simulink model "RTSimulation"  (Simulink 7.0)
settings: Solver=FixedStepDiscrete  StartTime=0.0  StopTime=inf  RelTol=1e-3
PreLoadFcn:
  | initialize;
  | scramInitialize;
InitFcn:
  | dirName = [bdroot '_xpc_rtw'];
  | if ~isdir(dirName)
  | 	mkdir(dirName);
  | end
  | copyfile('Actuator.obj', dirName);
  | copyfile('Act2Tbl.obj', dirName);
  | copyfile('Tbl2Act.obj', dirName);
  | copyfile('xfmlib.obj', dirName);
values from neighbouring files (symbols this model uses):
  acal = acal(:)    [initialize.m]
  actParams = [	bulkModulus   * pressCanon    [initialize.m]
  atype = ones(nact, 1)    [dampmatrix.m]    (also in displA2T.m = []; displEnvelope.m = varargin{1}{6}; displJacobian.m; displT2A.m = [])
  controlPeriod = 1/2048    (= 0.00048828125)    [initialize.m]
  dcal = dcal(:)    [initialize.m]
  fcal = fcal(:)    [initialize.m]
  forceCanon = 0.00444822    [initialize.m]
  inertia = inertia + inertiaP2Q([0 0 0], massA(i), cgA(:,i)-cg,  									inertiaCanon, massCanon)    [initialize.m]
  inertiaMask = zeros(3, 1)    [initialize.m]
  lengthCanon = 25.4    [initialize.m]
  mass = ones(3, 1) * (sum(massA) + massT + massS)    [initialize.m]
  massMask = zeros(3, 1)    [initialize.m]
  nAdcU = 6    [initialize.m]
  node = scgtnodestruct(node)    [scramInitialize.m]
  nTbl = length(dof)    [initialize.m]
  returnPress = 50    [initialize.m]
  rtg = cg    [initialize.m]
  samplePeriod = controlPeriod/upsampleFactor    (= 0.00048828125)    [initialize.m]    (also in viewer.m = eval(getHeaderValue(header, 'DELTA_T')))
  staticForce = forceT2A(ftbl, dtbl0, dof, rh, rb, rl, canon, atype)    [initialize.m]
  x = []    [loadbin.m]    (also in quake.m = 365; viewer.m = 40; player.m = xPanel + panelWide + margin; resondemo.m = xOrigin + marginWide + panelWide + plotMarginWide)
undefined symbols (not defined in the file or in its folder): animation, DiscIntNeverNeededParam, friction, yieldDispl
libraries: LibDynamics x12, LibTransforms x12, cwcec_scgtLib x3, xpclib x3

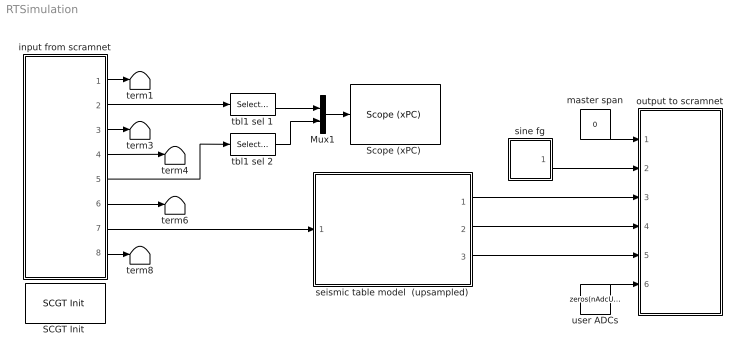
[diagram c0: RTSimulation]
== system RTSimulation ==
  Mux1 : Mux  Inputs=2
  "SCGT Init " : cwcec_scgtLib/SCGT Init   node=node  pci=-1
  "Scope (xPC) " : xpclib/Misc./Scope (xPC)   SystemSampleTime=-1  scopeno=1  scopetype=Target  autostart=on  viewmode=Graphical redraw  formatstr='%15.6f'  grid=on  ylimits=[0,0]  nosamples=1024  noprepostsamples=0  interleave=1  triggermode=FreeRun  triggersignal=1  triggerlevel=0.0  triggerslope=Either  triggerscope=1  triggersample=0  filename=data.dat  mode=Lazy  writesize=512  autorestart=off
  input from scramnet : Subsystem
  master span : Constant  Value=0  OutDataType=sfix(16)  OutScaling=2^0
  output to scramnet : Subsystem
  seismic table model  (upsampled) : Subsystem  TreatAsAtomicUnit=on
  sine fg : Subsystem  mask(Sine Function Generator){id=x, ampl=0.3, freq=4, phase=0, spanInterval=1, samplePeriod=controlPeriod}
      mask prompts: id "DOF"; ampl "Amplitude"; freq "Frequency (Hz)"; phase "Phase (deg)"; spanInterval "Span interval (sec)"; samplePeriod "Sample period (sec)"
  tbl1 sel 1 : Selector  IndexOptions=Index vector (dialog)  Indices=1  OutputSizes=1
  tbl1 sel 2 : Selector  IndexOptions=Index vector (dialog)  Indices=1  OutputSizes=1
  term{1,3..4,6,8} (5 alike) : Terminator
  user ADCs : Constant  Value=zeros(nAdcU, 1)  OutDataType=sfix(16)  OutScaling=2^0
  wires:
  input from scramnet/1(master span) -> term1/1
  input from scramnet/3(displ fbk) -> term3/1
  input from scramnet/4(veloc fbk) -> term4/1
  input from scramnet/6(force fbk) -> term6/1
  input from scramnet/8(user adcs) -> term8/1
  Mux1/1 -> "Scope (xPC) "/1
  input from scramnet/2(ref) -> tbl1 sel 1/1
  input from scramnet/5(accel fbk) -> tbl1 sel 2/1
  tbl1 sel 1/1 -> Mux1/1
  tbl1 sel 2/1 -> Mux1/2
  user ADCs/1 -> output to scramnet/6(user adcs)
  master span/1 -> output to scramnet/1(master span)
  input from scramnet/7(valve cmd) -> seismic table model  (upsampled)/1(valve cmd)
  sine fg/1(out) -> output to scramnet/2(ref)
  seismic table model  (upsampled)/1(displ) -> output to scramnet/3(displ fbk)
  seismic table model  (upsampled)/2(accel) -> output to scramnet/4(accel fbks)
  seismic table model  (upsampled)/3(force) -> output to scramnet/5(force fbk)

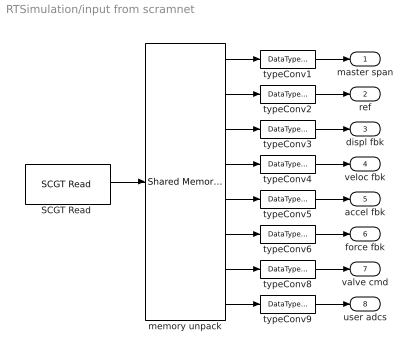
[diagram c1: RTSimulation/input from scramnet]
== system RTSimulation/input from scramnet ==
  "SCGT Read " : cwcec_scgtLib/SCGT Read   partition=node.Partitions(7:14)  ts=controlPeriod  pci=-1
  memory unpack : xpclib/Shared Memory/Shared Memory Unpack   partition=node.Partitions(7:14)
  typeConv{1..6,8..9} (8 alike) : DataTypeConversion  OutDataTypeMode=double  OutDataType=sfix(16)  OutScaling=2^0
  master span : Outport  OutDataType=sfix(16)  OutScaling=2^0
  ref : Outport  Port=2  OutDataType=sfix(16)  OutScaling=2^0
  displ fbk : Outport  Port=3  OutDataType=sfix(16)  OutScaling=2^0
  veloc fbk : Outport  Port=4  OutDataType=sfix(16)  OutScaling=2^0
  accel fbk : Outport  Port=5  OutDataType=sfix(16)  OutScaling=2^0
  force fbk : Outport  Port=6  OutDataType=sfix(16)  OutScaling=2^0
  valve cmd : Outport  Port=7  OutDataType=sfix(16)  OutScaling=2^0
  user adcs : Outport  Port=8  OutDataType=sfix(16)  OutScaling=2^0
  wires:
  "SCGT Read "/1 -> memory unpack/1
  typeConv1/1 -> master span/1
  typeConv2/1 -> ref/1
  typeConv3/1 -> displ fbk/1
  typeConv4/1 -> veloc fbk/1
  typeConv5/1 -> accel fbk/1
  typeConv6/1 -> force fbk/1
  typeConv8/1 -> valve cmd/1
  typeConv9/1 -> user adcs/1
  memory unpack/1 -> typeConv1/1
  memory unpack/8 -> typeConv9/1
  memory unpack/2 -> typeConv2/1
  memory unpack/7 -> typeConv8/1
  memory unpack/3 -> typeConv3/1
  memory unpack/4 -> typeConv4/1
  memory unpack/5 -> typeConv5/1
  memory unpack/6 -> typeConv6/1

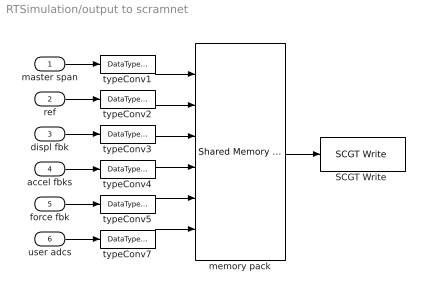
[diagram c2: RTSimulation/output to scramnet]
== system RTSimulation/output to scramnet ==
  master span : Inport  OutDataType=sfix(16)  OutScaling=2^0
  ref : Inport  Port=2  OutDataType=sfix(16)  OutScaling=2^0
  displ fbk : Inport  Port=3  OutDataType=sfix(16)  OutScaling=2^0
  accel fbks : Inport  Port=4  OutDataType=sfix(16)  OutScaling=2^0
  force fbk : Inport  Port=5  OutDataType=sfix(16)  OutScaling=2^0
  user adcs : Inport  Port=6  OutDataType=sfix(16)  OutScaling=2^0
  "SCGT Write " : cwcec_scgtLib/SCGT Write   partition=node.Partitions(1:6)  ts=controlPeriod  pci=-1
  memory pack : xpclib/Shared Memory/Shared Memory Pack   partition=node.Partitions(1:6)
  typeConv{1..5,7} (6 alike) : DataTypeConversion  OutDataTypeMode=single  OutDataType=sfix(16)  OutScaling=2^0
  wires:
  master span/1 -> typeConv1/1
  ref/1 -> typeConv2/1
  displ fbk/1 -> typeConv3/1
  accel fbks/1 -> typeConv4/1
  memory pack/1 -> "SCGT Write "/1
  typeConv1/1 -> memory pack/1
  typeConv2/1 -> memory pack/2
  typeConv3/1 -> memory pack/3
  typeConv4/1 -> memory pack/4
  force fbk/1 -> typeConv5/1
  user adcs/1 -> typeConv7/1
  typeConv5/1 -> memory pack/5
  typeConv7/1 -> memory pack/6

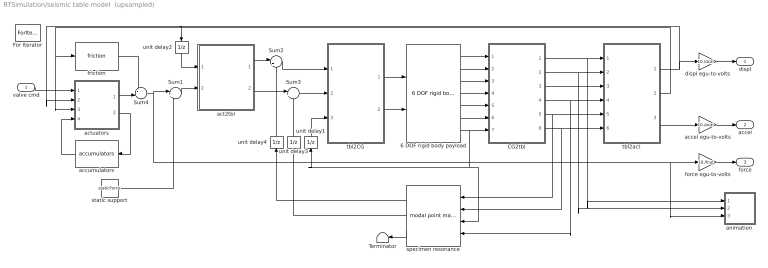
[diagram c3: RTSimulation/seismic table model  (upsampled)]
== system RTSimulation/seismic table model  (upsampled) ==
  valve cmd : Inport  OutDataType=sfix(16)  OutScaling=2^0
  6 DOF rigid body payload : LibDynamics/6 DOF rigid body payload  SystemSampleTime=-1  mass=mass.*massMask  inertia=diag(inertia.*inertiaMask)  gee=gee  massCanon=massCanon  inertiaCanon=inertiaCanon  linVelocCanon=linVelocCanon  linAccelCanon=linAccelCanon  rotDisplCanon=rotDisplCanon  rotVelocCanon=rotVelocCanon  rotAccelCanon=rotAccelCanon  rotForceCanon=rotForceCanon  initialPosition=zeros(6,1)  samplePeriod=samplePeriod
  CG2tbl : Subsystem  mask{ofst=-rtg}
      mask prompts: ofst "Origin offset"
  For Iterator : ForIterator  IterationLimit=upsampleFactor  ShowIterationPort=off
  Sum1 : Sum  Inputs=|++  OutDataType=sfix(16)  OutScaling=2^0
  Sum2 : Sum  Inputs=|+-  OutDataType=sfix(16)  OutScaling=2^0
  Sum3 : Sum  Inputs=|+-  OutDataType=sfix(16)  OutScaling=2^0
  Sum4 : Sum  Inputs=-+|  OutDataType=sfix(16)  OutScaling=2^0
  Terminator : Terminator
  accel egu-to-volts : Gain  Gain=10./acal  ParameterDataType=sfix(16)  ParameterScaling=2^0  OutDataType=sfix(16)  OutScaling=2^0
  accumulators : LibDynamics/accumulators  Orientation=left  SystemSampleTime=-1  pumpFlow=pumpFlow  supplyPressure=supplyPress  precharge=precharge  bottleVolume=volume  gasConstant=gasConstant  flowCanon=flowCanon  volumeCanon=volumeCanon  samplePeriod=samplePeriod
  act2tbl : Subsystem
  actuators : Subsystem
  animation : Subsystem  mask{azim=-37.5, elev=35, params=animation, decim=ceil((1/samplePeriod)/32), samplePeriod=-1}
      mask prompts: azim "View azimuth (degrees)"; elev "View elevation (degrees)"; params "Parameters"; decim "Decimation factor"; samplePeriod "Sample period (sec)"
  displ egu-to-volts : Gain  Gain=10./dcal  ParameterDataType=sfix(16)  ParameterScaling=2^0  OutDataType=sfix(16)  OutScaling=2^0
  force egu-to-volts : Gain  Gain=10./fcal  ParameterDataType=sfix(16)  ParameterScaling=2^0  OutDataType=sfix(16)  OutScaling=2^0
  friction : LibDynamics/friction  SystemSampleTime=-1  friction=friction * forceCanon  yieldDispl=yieldDispl * lengthCanon  hysteresis=0  velocCanon=linVelocCanon  samplePeriod=samplePeriod
  specimen resonance : LibDynamics/modal point mass  Orientation=left  SystemSampleTime=-1  mass=modalMass  freq=modalFreq  damp=modalDamp  ofst=modalCG  gee=gee  massCanon=massCanon  linAccelCanon=linAccelCanon  rotDisplCanon=rotDisplCanon  rotVelocCanon=rotVelocCanon  rotForceCanon=rotForceCanon  samplePeriod=samplePeriod
  static support : Constant  Value=staticForce  OutDataType=sfix(16)  OutScaling=2^0
  tbl2CG : Subsystem  mask{ofst=rtg}
      mask prompts: ofst "Origin offset"
  tbl2act : Subsystem
  unit delay1 : UnitDelay  Orientation=up  X0=eye(3)  SampleTime=-1
  unit delay2 : UnitDelay  Orientation=down  SampleTime=-1
  unit delay3 : UnitDelay  Orientation=up  SampleTime=-1
  unit delay4 : UnitDelay  Orientation=up  SampleTime=-1
  displ : Outport  OutDataType=sfix(16)  OutScaling=2^0
  accel : Outport  Port=2  OutDataType=sfix(16)  OutScaling=2^0
  force : Outport  Port=3  OutDataType=sfix(16)  OutScaling=2^0
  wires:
  specimen resonance/3 -> Terminator/1
  static support/1 -> Sum1/2
  Sum1/1 -> act2tbl/2(force act)
  accel egu-to-volts/1 -> accel/1
  displ egu-to-volts/1 -> displ/1
  force egu-to-volts/1 -> force/1
  accumulators/1 -> actuators/4(press)
  actuators/2(flow) -> accumulators/1
  tbl2CG/2(force rpw) -> 6 DOF rigid body payload/2
  tbl2act/1(displ act) -> displ egu-to-volts/1, actuators/2(displ), unit delay2/1
  valve cmd/1 -> actuators/1(cmds)
  tbl2CG/1(force xyz) -> 6 DOF rigid body payload/1
  6 DOF rigid body payload/1 -> CG2tbl/1(displ xyz)
  6 DOF rigid body payload/2 -> CG2tbl/2(displ rpw)
  6 DOF rigid body payload/3 -> CG2tbl/3(veloc xyz)
  6 DOF rigid body payload/4 -> CG2tbl/4(veloc rpw)
  6 DOF rigid body payload/5 -> CG2tbl/5(accel xyz)
  6 DOF rigid body payload/6 -> CG2tbl/6(accel rpw)
  6 DOF rigid body payload/7 -> specimen resonance/3, unit delay1/1, CG2tbl/7(DCM)
  tbl2act/3(accel act) -> accel egu-to-volts/1
  unit delay1/1 -> tbl2CG/3(DCM)
  unit delay2/1 -> act2tbl/1(displ act)
  tbl2act/2(veloc act) -> friction/1, actuators/3(veloc)
  CG2tbl/1(xyz) -> animation/1(xyz), tbl2act/1(xyz)
  CG2tbl/2(rpw) -> animation/2(rpw), tbl2act/2(rpw)
  CG2tbl/3(Vxyz) -> tbl2act/3(Vxyz)
  CG2tbl/4(Vrpw) -> specimen resonance/4, tbl2act/4(Vrpw)
  CG2tbl/5(Axyz) -> specimen resonance/1, tbl2act/5(Axyz)
  CG2tbl/6(Arpw) -> specimen resonance/2, tbl2act/6(Arpw)
  unit delay3/1 -> Sum3/2
  unit delay4/1 -> Sum2/2
  act2tbl/1(Fxyz) -> Sum2/1
  Sum2/1 -> tbl2CG/1(Fxyz)
  act2tbl/2(Frpw) -> Sum3/1
  Sum3/1 -> tbl2CG/2(Frpw)
  specimen resonance/1 -> unit delay4/1
  specimen resonance/2 -> unit delay3/1
  friction/1 -> Sum4/1
  actuators/1(force) -> Sum4/2
  Sum4/1 -> animation/3(Fact), force egu-to-volts/1, Sum1/1

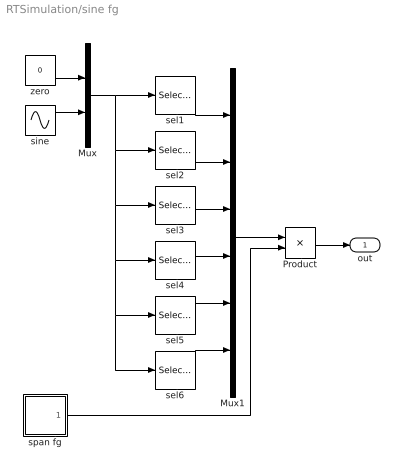
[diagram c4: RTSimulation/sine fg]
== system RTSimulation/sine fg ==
  Mux : Mux  Inputs=2
  Mux1 : Mux  Inputs=6
  Product : Product  OutDataType=sfix(16)  OutScaling=2^0
  sel1 : Selector  InputPortWidth=2  IndexOptions=Index vector (dialog)  Indices=(id==1)+1  OutputSizes=1
  sel2 : Selector  InputPortWidth=2  IndexOptions=Index vector (dialog)  Indices=(id==2)+1  OutputSizes=1
  sel3 : Selector  InputPortWidth=2  IndexOptions=Index vector (dialog)  Indices=(id==3)+1  OutputSizes=1
  sel4 : Selector  InputPortWidth=2  IndexOptions=Index vector (dialog)  Indices=(id==4)+1  OutputSizes=1
  sel5 : Selector  InputPortWidth=2  IndexOptions=Index vector (dialog)  Indices=(id==5)+1  OutputSizes=1
  sel6 : Selector  InputPortWidth=2  IndexOptions=Index vector (dialog)  Indices=(id==6)+1  OutputSizes=1
  sine : Sin  Amplitude=ampl  Frequency=2 * pi * freq  Phase=phase*180/pi  SampleTime=samplePeriod
  span fg : Subsystem  mask{spanInterval=spanInterval, samplePeriod=samplePeriod}
      mask prompts: spanInterval "Span interval (sec)"; samplePeriod "Sample period (sec)"
  zero : Constant  Value=0  OutDataType=sfix(16)  OutScaling=2^0  SampleTime=samplePeriod
  out : Outport  OutDataType=sfix(16)  OutScaling=2^0
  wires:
  span fg/1(out) -> Product/2
  Product/1 -> out/1
  Mux1/1 -> Product/1
  zero/1 -> Mux/1
  sine/1 -> Mux/2
  sel1/1 -> Mux1/1
  sel2/1 -> Mux1/2
  sel3/1 -> Mux1/3
  sel4/1 -> Mux1/4
  sel5/1 -> Mux1/5
  sel6/1 -> Mux1/6
  Mux/1 -> sel2/1, sel3/1, sel4/1, sel5/1, sel6/1, sel1/1

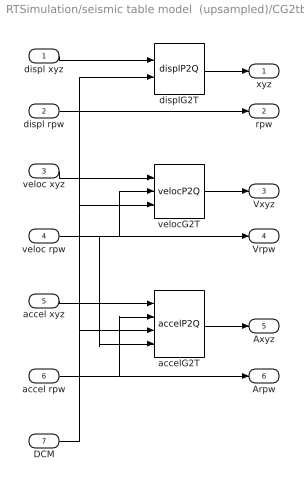
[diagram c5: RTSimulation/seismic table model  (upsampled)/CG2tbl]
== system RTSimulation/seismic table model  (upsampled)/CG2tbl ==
  displ xyz : Inport  OutDataType=sfix(16)  OutScaling=2^0
  displ rpw : Inport  Port=2  OutDataType=sfix(16)  OutScaling=2^0
  veloc xyz : Inport  Port=3  OutDataType=sfix(16)  OutScaling=2^0
  veloc rpw : Inport  Port=4  OutDataType=sfix(16)  OutScaling=2^0
  accel xyz : Inport  Port=5  OutDataType=sfix(16)  OutScaling=2^0
  accel rpw : Inport  Port=6  OutDataType=sfix(16)  OutScaling=2^0
  DCM : Inport  Port=7  OutDataType=sfix(16)  OutScaling=2^0
  accelG2T : LibTransforms/accelP2Q  SystemSampleTime=-1  dof=1:6  ofst=ofst
  displG2T : LibTransforms/displP2Q  SystemSampleTime=-1  dof=1:6  ofst=ofst
  velocG2T : LibTransforms/velocP2Q  SystemSampleTime=-1  dof=1:6  ofst=ofst
  xyz : Outport  OutDataType=sfix(16)  OutScaling=2^0
  rpw : Outport  Port=2  OutDataType=sfix(16)  OutScaling=2^0
  Vxyz : Outport  Port=3  OutDataType=sfix(16)  OutScaling=2^0
  Vrpw : Outport  Port=4  OutDataType=sfix(16)  OutScaling=2^0
  Axyz : Outport  Port=5  OutDataType=sfix(16)  OutScaling=2^0
  Arpw : Outport  Port=6  OutDataType=sfix(16)  OutScaling=2^0
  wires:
  accel rpw/1 -> accelG2T/2, Arpw/1
  DCM/1 -> accelG2T/3, velocG2T/3, displG2T/2
  veloc rpw/1 -> accelG2T/4, velocG2T/2, Vrpw/1
  veloc xyz/1 -> velocG2T/1
  accel xyz/1 -> accelG2T/1
  displ xyz/1 -> displG2T/1
  displG2T/1 -> xyz/1
  displ rpw/1 -> rpw/1
  velocG2T/1 -> Vxyz/1
  accelG2T/1 -> Axyz/1

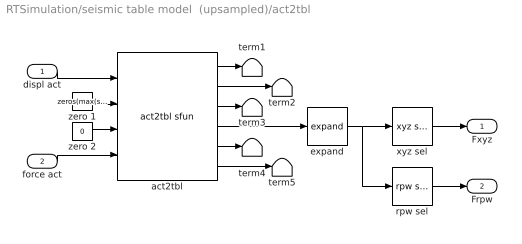
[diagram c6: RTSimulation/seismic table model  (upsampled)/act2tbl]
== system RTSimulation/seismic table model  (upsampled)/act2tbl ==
  displ act : Inport  OutDataType=sfix(16)  OutScaling=2^0
  force act : Inport  Port=2  OutDataType=sfix(16)  OutScaling=2^0
  act2tbl : LibTransforms/act2tbl sfun  atype=atype  nVel=0  nFrc=length(atype)  dof=dof  rh=rh  rb=rb  rl=rl  ra=[]  ea=[]  offset=[0 0 0 0 0 0]  dmax=dmax  fmax=fmax  canon=canon  gee=gee  action=1  rate=0  count=1
  expand : LibTransforms/expand  SystemSampleTime=-1  size=6  elements=dof
  rpw sel : LibTransforms/rpw sel  SystemSampleTime=-1  dof=1:6
  term{1..5} (5 alike) : Terminator
  xyz sel : LibTransforms/xyz sel  SystemSampleTime=-1  dof=1:6
  zero 1 : Constant  Value=zeros(max(sum(dof>3), 1), 1)  OutDataType=sfix(16)  OutScaling=2^0
  zero 2 : Constant  Value=0  OutDataType=sfix(16)  OutScaling=2^0
  Fxyz : Outport  OutDataType=sfix(16)  OutScaling=2^0
  Frpw : Outport  Port=2  OutDataType=sfix(16)  OutScaling=2^0
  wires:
  rpw sel/1 -> Frpw/1
  force act/1 -> act2tbl/4
  xyz sel/1 -> Fxyz/1
  displ act/1 -> act2tbl/1
  act2tbl/4 -> expand/1
  zero 2/1 -> act2tbl/3
  zero 1/1 -> act2tbl/2
  act2tbl/1 -> term1/1
  act2tbl/2 -> term2/1
  act2tbl/3 -> term3/1
  act2tbl/5 -> term4/1
  act2tbl/6 -> term5/1
  expand/1 -> rpw sel/1, xyz sel/1

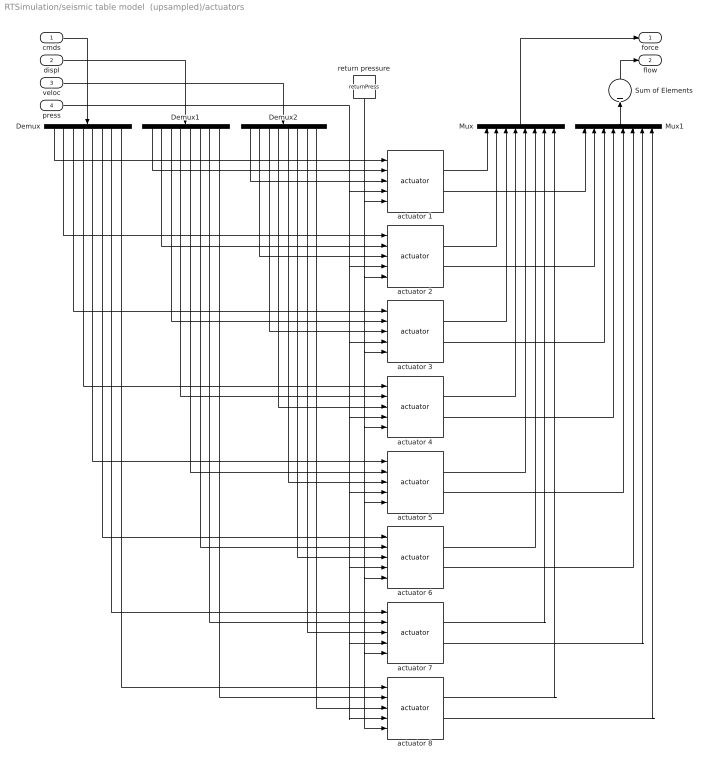
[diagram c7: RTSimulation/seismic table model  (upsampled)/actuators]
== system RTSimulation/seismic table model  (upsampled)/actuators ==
  cmds : Inport  OutDataType=sfix(16)  OutScaling=2^0
  displ : Inport  Port=2  OutDataType=sfix(16)  OutScaling=2^0
  veloc : Inport  Port=3  OutDataType=sfix(16)  OutScaling=2^0
  press : Inport  Port=4  OutDataType=sfix(16)  OutScaling=2^0
  Demux : Demux  Orientation=down  Outputs=nAct
  Demux1 : Demux  Orientation=down  Outputs=nAct
  Demux2 : Demux  Orientation=down  Outputs=nAct
  Mux : Mux  Orientation=up  Inputs=nAct
  Mux1 : Mux  Orientation=up  Inputs=nAct
  Sum of Elements : Sum  Orientation=up  Inputs=+  OutDataType=sfix(16)  OutScaling=2^-10
  actuator 1 : LibDynamics/actuator  SystemSampleTime=-1  params=actParams(:,1)
  actuator 2 : LibDynamics/actuator  SystemSampleTime=-1  params=actParams(:,2)
  actuator 3 : LibDynamics/actuator  SystemSampleTime=-1  params=actParams(:,3)
  actuator 4 : LibDynamics/actuator  SystemSampleTime=-1  params=actParams(:,4)
  actuator 5 : LibDynamics/actuator  SystemSampleTime=-1  params=actParams(:,5)
  actuator 6 : LibDynamics/actuator  SystemSampleTime=-1  params=actParams(:,6)
  actuator 7 : LibDynamics/actuator  SystemSampleTime=-1  params=actParams(:,7)
  actuator 8 : LibDynamics/actuator  SystemSampleTime=-1  params=actParams(:,8)
  return pressure : Constant  Orientation=down  Value=returnPress  OutDataType=sfix(16)  OutScaling=2^0
  force : Outport  OutDataType=sfix(16)  OutScaling=2^0
  flow : Outport  Port=2  OutDataType=sfix(16)  OutScaling=2^0
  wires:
  Mux/1 -> force/1
  cmds/1 -> Demux/1
  displ/1 -> Demux1/1
  Demux/1 -> actuator 1/1
  Demux/2 -> actuator 2/1
  Demux1/1 -> actuator 1/2
  Demux2/1 -> actuator 1/3
  Demux1/2 -> actuator 2/2
  Demux2/2 -> actuator 2/3
  Demux/3 -> actuator 3/1
  Demux1/3 -> actuator 3/2
  Demux2/3 -> actuator 3/3
  Demux/4 -> actuator 4/1
  Demux1/4 -> actuator 4/2
  Demux2/4 -> actuator 4/3
  Demux/5 -> actuator 5/1
  Demux1/5 -> actuator 5/2
  Demux2/5 -> actuator 5/3
  Demux/6 -> actuator 6/1
  Demux1/6 -> actuator 6/2
  Demux2/6 -> actuator 6/3
  Demux/7 -> actuator 7/1
  Demux1/7 -> actuator 7/2
  Demux2/7 -> actuator 7/3
  Demux/8 -> actuator 8/1
  Demux1/8 -> actuator 8/2
  Demux2/8 -> actuator 8/3
  actuator 1/1 -> Mux/1
  actuator 2/1 -> Mux/2
  actuator 3/1 -> Mux/3
  actuator 4/1 -> Mux/4
  actuator 5/1 -> Mux/5
  actuator 6/1 -> Mux/6
  actuator 7/1 -> Mux/7
  actuator 8/1 -> Mux/8
  veloc/1 -> Demux2/1
  press/1 -> actuator 7/4, actuator 8/4, actuator 6/4, actuator 5/4, actuator 4/4, actuator 3/4, actuator 2/4, actuator 1/4
  return pressure/1 -> actuator 7/5, actuator 8/5, actuator 6/5, actuator 5/5, actuator 4/5, actuator 3/5, actuator 2/5, actuator 1/5
  Mux1/1 -> Sum of Elements/1
  actuator 1/2 -> Mux1/1
  actuator 2/2 -> Mux1/2
  actuator 3/2 -> Mux1/3
  actuator 4/2 -> Mux1/4
  actuator 5/2 -> Mux1/5
  actuator 6/2 -> Mux1/6
  actuator 7/2 -> Mux1/7
  actuator 8/2 -> Mux1/8
  Sum of Elements/1 -> flow/1

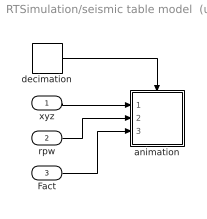
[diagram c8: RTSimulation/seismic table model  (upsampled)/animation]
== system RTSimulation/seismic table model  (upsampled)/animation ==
  xyz : Inport
  rpw : Inport  Port=2
  Fact : Inport  Port=3
  animation : Subsystem  TreatAsAtomicUnit=on
  decimation : DiscretePulseGenerator  Period=decim  SampleTime=samplePeriod
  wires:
  decimation/1 -> animation/Trigger
  xyz/1 -> animation/1(xyz)
  Fact/1 -> animation/3(Fact)
  rpw/1 -> animation/2(rpw)

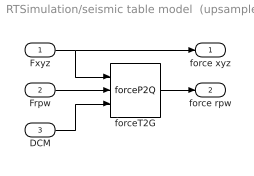
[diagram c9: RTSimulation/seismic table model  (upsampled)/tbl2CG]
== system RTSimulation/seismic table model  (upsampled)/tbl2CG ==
  Fxyz : Inport  OutDataType=sfix(16)  OutScaling=2^0
  Frpw : Inport  Port=2  OutDataType=sfix(16)  OutScaling=2^0
  DCM : Inport  Port=3  OutDataType=sfix(16)  OutScaling=2^0
  forceT2G : LibTransforms/forceP2Q  SystemSampleTime=-1  dof=1:6  ofst=ofst
  force xyz : Outport  OutDataType=sfix(16)  OutScaling=2^0
  force rpw : Outport  Port=2  OutDataType=sfix(16)  OutScaling=2^0
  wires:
  DCM/1 -> forceT2G/3
  forceT2G/1 -> force rpw/1
  Fxyz/1 -> force xyz/1, forceT2G/1
  Frpw/1 -> forceT2G/2

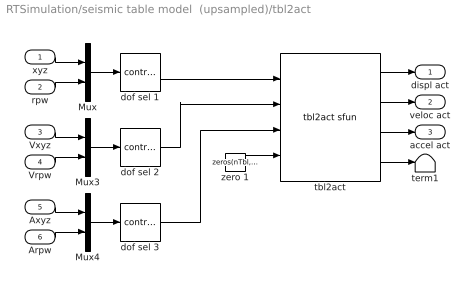
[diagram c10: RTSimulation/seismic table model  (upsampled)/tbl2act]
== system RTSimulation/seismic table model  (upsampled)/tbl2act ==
  xyz : Inport  OutDataType=sfix(16)  OutScaling=2^0
  rpw : Inport  Port=2  OutDataType=sfix(16)  OutScaling=2^0
  Vxyz : Inport  Port=3  OutDataType=sfix(16)  OutScaling=2^0
  Vrpw : Inport  Port=4  OutDataType=sfix(16)  OutScaling=2^0
  Axyz : Inport  Port=5  OutDataType=sfix(16)  OutScaling=2^0
  Arpw : Inport  Port=6  OutDataType=sfix(16)  OutScaling=2^0
  Mux : Mux  Inputs=2
  Mux3 : Mux  Inputs=2
  Mux4 : Mux  Inputs=2
  dof sel 1 : LibTransforms/contract  SystemSampleTime=-1  elements=dof
  dof sel 2 : LibTransforms/contract  SystemSampleTime=-1  elements=dof
  dof sel 3 : LibTransforms/contract  SystemSampleTime=-1  elements=dof
  tbl2act : LibTransforms/tbl2act sfun  atype=atype  nVel=length(atype)  nFrc=0  dof=dof  rh=rh  rb=rb  rl=rl  ra=ra  ea=ea  offset=[0 0 0 0 0 0]  fmax=fmax  canon=canon  gee=gee  action=1  rate=0
  term1 : Terminator
  zero 1 : Constant  Value=zeros(nTbl, 1)  OutDataType=sfix(16)  OutScaling=2^0
  displ act : Outport  OutDataType=sfix(16)  OutScaling=2^0
  veloc act : Outport  Port=2  OutDataType=sfix(16)  OutScaling=2^0
  accel act : Outport  Port=3  OutDataType=sfix(16)  OutScaling=2^0
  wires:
  Mux4/1 -> dof sel 3/1
  Mux3/1 -> dof sel 2/1
  Mux/1 -> dof sel 1/1
  Arpw/1 -> Mux4/2
  Axyz/1 -> Mux4/1
  Vrpw/1 -> Mux3/2
  Vxyz/1 -> Mux3/1
  rpw/1 -> Mux/2
  xyz/1 -> Mux/1
  zero 1/1 -> tbl2act/4
  tbl2act/4 -> term1/1
  tbl2act/3 -> accel act/1
  tbl2act/2 -> veloc act/1
  tbl2act/1 -> displ act/1
  dof sel 1/1 -> tbl2act/1
  dof sel 2/1 -> tbl2act/2
  dof sel 3/1 -> tbl2act/3

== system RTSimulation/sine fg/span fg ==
  integrator : DiscreteIntegrator  SampleTime=samplePeriod  OutDataType=sfix(16)  OutScaling=2^0  LimitOutput=on  UpperSaturationLimit=1  LowerSaturationLimit=0  ICPrevOutput=DiscIntNeverNeededParam  ICPrevScaledInput=DiscIntNeverNeededParam
  span rate : Constant  Value=1/max(spanInterval,samplePeriod)  OutDataType=sfix(16)  OutScaling=2^0  SampleTime=samplePeriod
  out : Outport  OutDataType=sfix(16)  OutScaling=2^0
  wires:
  span rate/1 -> integrator/1
  integrator/1 -> out/1

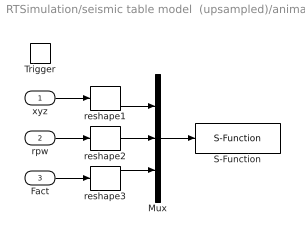
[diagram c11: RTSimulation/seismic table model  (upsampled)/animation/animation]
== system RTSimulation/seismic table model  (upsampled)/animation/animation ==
  xyz : Inport  OutDataType=sfix(16)  OutScaling=2^0
  rpw : Inport  Port=2  OutDataType=sfix(16)  OutScaling=2^0
  Fact : Inport  Port=3  OutDataType=sfix(16)  OutScaling=2^0
  Trigger : TriggerPort
  Mux : Mux  Inputs=3
  S-Function : S-Function  FunctionName=animation  Parameters=azim,elev,params
  reshape1 : Reshape
  reshape2 : Reshape
  reshape3 : Reshape
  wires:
  Mux/1 -> S-Function/1
  xyz/1 -> reshape1/1
  Fact/1 -> reshape3/1
  reshape3/1 -> Mux/3
  rpw/1 -> reshape2/1
  reshape2/1 -> Mux/2
  reshape1/1 -> Mux/1
